// ********************************************************************************

TYPE UDT 71

  STRUCT
   IFNo : ARRAY  [1 .. 16 ] OF BOOL ;   //Interface [no.] active
   Quit : ARRAY  [1 .. 16 ] OF BOOL ;   //perform Quit-End
   IF : ARRAY  [1 .. 16 ] OF STRUCT
    Loading : BOOL ;
    Unloading : BOOL ;
    Reloading : BOOL ;
    Positioning : BOOL ;
    PosbyProgram : BOOL ;   //Initiation by CNC Program
    PositioningMT : BOOL ;  //Positioning Multitool
    f0_6 : BOOL ;
    f0_7 : BOOL ;
    PerfStatusError : BOOL ;
    n1_1 : BOOL ;
    n1_2 : BOOL ;
    n1_3 : BOOL ;
    n1_4 : BOOL ;
    n1_5 : BOOL ;
    n1_6 : BOOL ;
    DataInDB1071 : BOOL ;
    Channel : BYTE ;    //Assigned channel
    TMno : BYTE ;   //Tool management no.
    Free1 : DINT ;  //Unassigned parameter 1
    Free2 : DINT ;  //Unassigned parameter 2
    Free3 : DINT ;  //Unassigned parameter 3
    IdentLoad : INT ;   //Identification for loading/unloading station
    NoLoad : INT ;  //No. of loading station
    SMag : INT ;    //Magazine no. (source) for unloading/reloading/pos.
    SLoc : INT ;    //Location no. (source) for unloading/reloading/pos.
    TMag : INT ;    //Magazine no. (target) for loading/reloading
    TLoc : INT ;    //Location no. (target) for loading/reloading
    WithoutMagMoving : BOOL ;   //HMI Data: Without Magazine Moving
    Res2 : BYTE ;
   END_STRUCT ;
  END_STRUCT ;
END_TYPE


// ********************************************************************************

TYPE UDT 72

  STRUCT
   IFNo : ARRAY  [1 .. 16 ] OF BOOL ;   //Interface [no.] active
   Quit : ARRAY  [1 .. 16 ] OF BOOL ;   //perform Quit-End
   IF : ARRAY  [1 .. 16 ] OF STRUCT
    Comp : BOOL ;   //Compulsory change
    Perform : BOOL ;    //Perform change
    Prepare : BOOL ;    //Prepare change
    T0 : BOOL ;     //T0 programmed
    OldTinDBW42 : BOOL ;    //ZWS No. of Old Tool in DBW (n+42)
    ManTIn : BOOL ; //Put in Tool in Spindle manual
    ManTOut : BOOL ;    //Get out Tool from Spindle manual
    SpiTRSpi : BOOL ;    //Spindle Tool remains in spindle
    PerfStatusError : BOOL ;
    n1_1 : BOOL ;
    n1_2 : BOOL ;
    n1_3 : BOOL ;
    n1_4 : BOOL ;
    n1_5 : BOOL ;
    n1_6 : BOOL ;
    DataInDB1072 : BOOL ;
    Channel : BYTE ;    //Assigned channel
    TMno : BYTE ;   //Tool management no.
    Free1 : DINT ;  //Unassigned parameter 1
    Free2 : DINT ;  //Unassigned parameter 2
    Free3 : DINT ;  //Unassigned parameter 3
    IdentBuff : INT ;   //Buffer identification (fixed value 9998)
    NoBuff : INT ;  //Relative location (target) in the buffer
    SMag : INT ;    //Magazine no. (source) for new tool
    SLoc : INT ;    //Location no. (source) for new tool
    TMag : INT ;    //Magazine no. (target) for old tool
    TLoc : INT ;    //Location no. (target) for old tool
    LocType : INT ; //Tool new: location type
    SLeft : INT ;   //Tool new: size left
    SRight : INT ;  //Tool new: size right
    STop : INT ;    //Tool new: size top
    SBottom : INT ; //Tool new: size bottom
    ToolInBuff : BOOL;  //ID for tools in buffer
    IgnoreDisab : BOOL; //Ignore disabled
    TBUnloaded : BOOL;  //To be unloaded
    TBLoaded : BOOL;    //To be loaded
    MasterTool : BOOL;  //Master tool
    n38_5 : BOOL;       //reserved
    Exchange_1to1 : BOOL; //1:1 exchange
    HandTool : BOOL;    //Hand tool
    ActTool : BOOL;     //Active tool
    ToolEnabl : BOOL;   //Tool enabled
    ToolDisab : BOOL;   //Tool disabled
    Measured : BOOL;    //Tool measured
    Prewarn : BOOL;     //Prewarning limit reached
    ToolChange : BOOL;  //Tool being changed
    FixedLoc : BOOL;    //Tool fixed location coded
    ToolUsed : BOOL;    //Tool was in use
    T_no : INT ;    //Tool new: T no.
    OldTZWSNo : INT ;   //ZWS No. of Old Tool
    MyMag : INT ;
    MyPlace : INT ;
   END_STRUCT ;
  END_STRUCT ;
END_TYPE


// ********************************************************************************

TYPE UDT 73

  STRUCT
   IfNo : ARRAY  [1 .. 16 ] OF BOOL ;   //Interface [no.] active
   Quit : ARRAY  [1 .. 16 ] OF BOOL ;   //perform Quit-End
   IF : ARRAY  [1 .. 16 ] OF STRUCT
    Comp : BOOL ;   //Compulsory change
    Perform : BOOL ;    //Perform change
    f0_2 : BOOL ;
    T0 : BOOL ;     //T0 programmed
    f0_4 : BOOL ;
    f0_5 : BOOL ;
    ManTOut : BOOL ;    //Get out Tool from Holder manual
    f0_7 : BOOL ;
    PerfStatusError : BOOL ;
    n1_1 : BOOL ;
    n1_2 : BOOL ;
    n1_3 : BOOL ;
    n1_4 : BOOL ;
    n1_5 : BOOL ;
    n1_6 : BOOL ;
    DataInDB1073 : BOOL ;
    Channel : BYTE ;    //Assigned channel
    TMno : BYTE ;   //Tool management no.
    Free1 : DINT ;  //Unassigned parameter 1
    Free2 : DINT ;  //Unassigned parameter 2
    Free3 : DINT ;  //Unassigned parameter 3
    KennZWS : INT ; //Reserved (buffer identification)
    NoBuff : INT ;  //Rel. location in buffer (res.)
    SMag : INT ;    //Magazine no. of turret
    SLoc : INT ;    //Location no. for new tool
    TMag : INT ;    //Magazine no. of turret (res.)
    TLoc : INT ;    //Location no. for old tool
    LocType : INT ; //Tool new: location type
    SLeft : INT ;   //Tool new: size left
    SRight : INT ;  //Tool new: size right
    STop : INT ;    //Tool new: size top
    SBottom : INT ; //Tool new: size bottom
    ToolInBuff : BOOL;  //ID for tools in buffer
    IgnoreDisab : BOOL; //Ignore disabled
    TBUnloaded : BOOL;  //To be unloaded
    TBLoaded : BOOL;    //To be loaded
    MasterTool : BOOL;  //Master tool
    n38_5 : BOOL;       //reserved
    Exchange_1to1 : BOOL; //1:1 exchange
    HandTool : BOOL;    //Hand tool
    ActTool : BOOL;     //Active tool
    ToolEnabl : BOOL;   //Tool enabled
    ToolDisab : BOOL;   //Tool disabled
    Measured : BOOL;    //Tool measured
    Prewarn : BOOL;     //Prewarning limit reached
    ToolChange : BOOL;  //Tool being changed
    FixedLoc : BOOL;    //Tool fixed location coded
    ToolUsed : BOOL;    //Tool was in use
    T_no : INT ;    //Tool new: T no.
    MyPlace : INT ;
   END_STRUCT ;
  END_STRUCT ;
END_TYPE


// ********************************************************************************

TYPE UDT 1071

  STRUCT
   MTIF : ARRAY  [1 .. 16 ] OF STRUCT
    MtType          : INT;
    MtPlaces        : INT;
    MtDistance      : REAL;
    MtNum           : INT ; // MT-No. to be positioned to
    MtPlaceNum      : INT ; // MT-PlaceNo. ~
    ToolHolder      : INT ; // TH-No as reference for MT-positioning

    IF : ARRAY  [1 .. 3 ] OF STRUCT
     reserved       : INT;  // reserved
    END_STRUCT ;

   END_STRUCT ;
  END_STRUCT ;
END_TYPE


// ********************************************************************************

TYPE UDT 1072

  STRUCT
   MTIF : ARRAY  [1 .. 16 ] OF STRUCT
    MtType          : INT;
    MtPlaces        : INT;
    MtDistance      : REAL;
    MtNumNew        : INT;  // MT-No. new Tool
    MtPlaceNumNew   : INT;  // MtoolPlaceNum  ~
    MtNumOld        : INT;  // MT-No. old Tool
    MtPlaceNumOld   : INT;  // MtoolPlaceNum  ~
    LocType : INT ; //Tool new: location type
    SLeft : INT ; //Tool new: size left
    SRight : INT ;  //Tool new: size right
    STop : INT ;  //Tool new: size top
    SBottom : INT ; //Tool new: size bottom

    ToolInBuff : BOOL;  //ID for tools in buffer
    IgnoreDisab : BOOL; //Ignore disabled
    TBUnloaded : BOOL;  //To be unloaded
    TBLoaded : BOOL;    //To be loaded
    MasterTool : BOOL;  //Master tool
    n26_5 : BOOL;       //reserved
    n26_6 : BOOL;       //reserved
    HandTool : BOOL;    //Hand tool

    ActTool : BOOL;     //Active tool
    ToolEnabl : BOOL;   //Tool enabled
    ToolDisab : BOOL;   //Tool disabled
    Measured : BOOL;    //Tool measured
    Prewarn : BOOL;     //Prewarning limit reached
    ToolChange : BOOL;  //Tool being changed
    FixedLoc : BOOL;    //Tool fixed location coded
    ToolUsed : BOOL;    //Tool was in use

    T_no : INT ;  //Tool new: T no.
    ToolHolder      : INT; // TH-No as tool compensation reference
    MtMyMag         : INT; // MtoolNumber the tool is loaded onto
    MtMyPlace       : INT; // MtoolPlaceNum ~

    IF : ARRAY  [1 .. 7 ] OF STRUCT
     reserved       : INT;  // reserved
    END_STRUCT ;

   END_STRUCT ;
  END_STRUCT ;
END_TYPE


// ********************************************************************************

TYPE UDT 1073

  STRUCT
   MTIF : ARRAY  [1 .. 16 ] OF STRUCT
    MtType          : INT;
    MtPlaces        : INT;
    MtDistance      : REAL;
    MtNumNew        : INT;  // MT-No. new Tool
    MtPlaceNumNew   : INT;  // MtoolPlaceNum  ~
    MtNumOld        : INT;  // MT-No. old Tool
    MtPlaceNumOld   : INT;  // MtoolPlaceNum  ~
    LocType : INT ; //Tool new: location type
    SLeft : INT ; //Tool new: size left
    SRight : INT ;  //Tool new: size right
    STop : INT ;  //Tool new: size top
    SBottom : INT ; //Tool new: size bottom

    ToolInBuff : BOOL;  //ID for tools in buffer
    IgnoreDisab : BOOL; //Ignore disabled
    TBUnloaded : BOOL;  //To be unloaded
    TBLoaded : BOOL;    //To be loaded
    MasterTool : BOOL;  //Master tool
    n26_5 : BOOL;       //reserved
    n26_6 : BOOL;       //reserved
    HandTool : BOOL;    //Hand tool

    ActTool : BOOL;     //Active tool
    ToolEnabl : BOOL;   //Tool enabled
    ToolDisab : BOOL;   //Tool disabled
    Measured : BOOL;    //Tool measured
    Prewarn : BOOL;     //Prewarning limit reached
    ToolChange : BOOL;  //Tool being changed
    FixedLoc : BOOL;    //Tool fixed location coded
    ToolUsed : BOOL;    //Tool was in use

    T_no : INT ;  //Tool new: T no.
    ToolHolder      : INT; // TH-No as tool compensation reference
    MtMyMag         : INT; // MtoolNumber the tool is loaded onto
    MtMyPlace       : INT; // MtoolPlaceNum ~

    IF : ARRAY  [1 .. 7 ] OF STRUCT
     reserved       : INT;  // reserved
    END_STRUCT ;

   END_STRUCT ;
  END_STRUCT ;
END_TYPE
